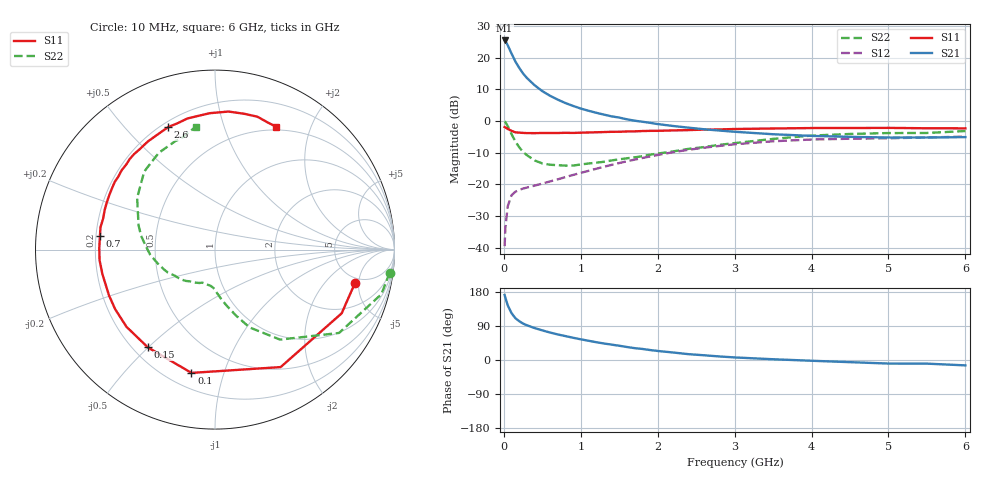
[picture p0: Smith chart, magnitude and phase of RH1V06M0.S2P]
! SIEMENS Small Signal Semiconductors
! BFR106
! Si NPN RF Bipolar Junction Transistor in SOT23
! VCE = 1 V  IC = 6 mA
! Common Emitter S-Parameters:  August  1996
# GHz  S  MA  R  50
!  f  S11  S21  S12  S22
! GHz  MAG  ANG  MAG  ANG  MAG  ANG  MAG  ANG
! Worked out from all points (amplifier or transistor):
!   36 points, 10 MHz to 6 GHz, reference 50 ohm
!   highest |S21| = 25.4 dB at 10 MHz (marker M1)
!   |S21| within 3 dB of that: start of sweep to 78.56 MHz
!   unconditionally stable (mu >= 1): 559.4 MHz to 2.89 GHz; 3.415 GHz to end of sweep
!   at 250 MHz: K = 0.57, MSG = 18.2 dB, |S12| = -21.4 dB
!   at 1.4 GHz: K = 1.17, MAG = 5.2 dB, |S12| = -13.9 dB
!   at 6 GHz: K = 1.03, MAG = -1.1 dB, |S12| = -5.0 dB
!   S11 on the Smith chart (normalised r, x): 10 MHz: 4.27, -4.47; 100 MHz: 0.29, -0.78; 150 MHz: 0.26, -0.50; 700 MHz: 0.22, +0.06; 2.6 GHz: 0.23, +0.66; 6 GHz: 0.46, +1.52
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0.01  0.8016 -13.5  18.73 171.5  0.0105 84.1  0.9817 -7.5
0.02  0.7901 -26.7  18.33 164.5  0.0204 76.3  0.9599 -15.0
0.05  0.7498 -60.8  15.8 144.5  0.0446 60.6  0.8327 -33.9
0.1  0.6994 -100.8  11.62 123.6  0.0669 45.3  0.6191 -54.1
0.15  0.6609 -124.5  8.709 110.4  0.0762 37.6  0.474 -66.1
0.2  0.6543 -138.9  6.907 102.4  0.0813 35.1  0.3847 -72.4
0.25  0.6477 -149.1  5.63 96.1  0.0855 34.3  0.323 -77.8
0.3  0.6434 -156.6  4.778 91.6  0.0886 35.1  0.288 -81.7
0.4  0.642 -167.7  3.668 84.3  0.0952 37.0  0.238 -88.0
0.5  0.6459 -174.8  2.961 78.2  0.1024 39.4  0.2132 -92.5
0.6  0.6447 179.1  2.502 72.5  0.1108 42.0  0.2034 -96.9
0.7  0.6456 173.3  2.177 67.5  0.1194 44.6  0.1999 -101.9
0.9  0.6467 164.6  1.729 58.7  0.1402 48.4  0.1973 -111.0
1.1  0.6579 156.4  1.451 50.8  0.1628 50.6  0.2125 -119.8
1.3  0.6678 149.2  1.261 43.6  0.1888 51.7  0.2262 -128.6
1.6  0.6825 139.7  1.062 34.3  0.2306 51.4  0.2571 -141.8
2.2  0.709 121.9  0.833 19.8  0.3208 45.5  0.3303 -167.0
2.6  0.7305 111.0  0.74 12.5  0.3776 39.4  0.3865 177.0
3.5  0.7605 92.3  0.617 2.0  0.4778 23.8  0.5209 146.4
4.5  0.774 77.9  0.561 -5.7  0.524 7.6  0.6234 120.2
5.5  0.7666 67.3  0.548 -9.6  0.5491 -2.0  0.6456 107.4
6  0.7644 63.5  0.556 -14.2  0.5652 -8.7  0.6933 98.8
